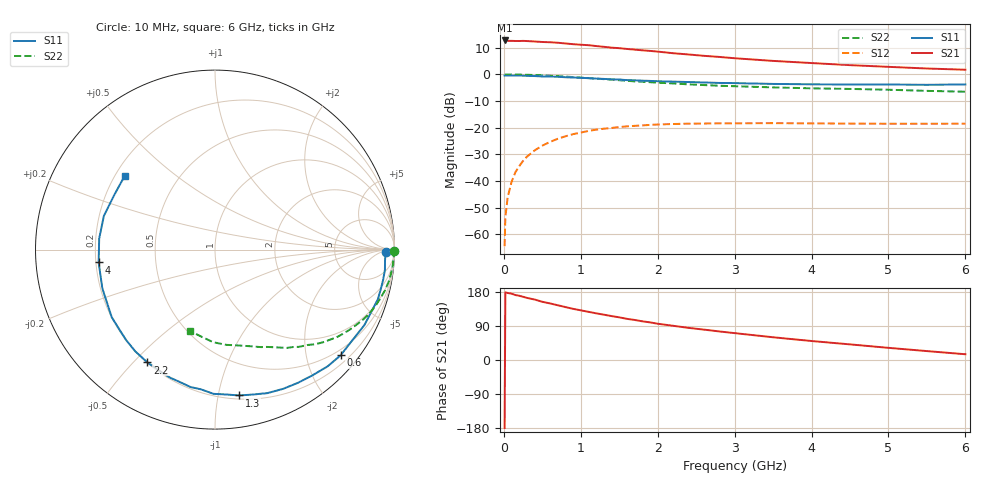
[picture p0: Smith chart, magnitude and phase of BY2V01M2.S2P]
! SIEMENS Small Signal Semiconductors
! BFY420
! Si NPN RF SIEGET Grounded Emitter Transistor in MICRO-X
! VCE = 2 V  IC = 1.2 mA
! Common Emitter S-Parameters:  October  1996
# GHz  S  MA  R  50
!  f  S11  S21  S12  S22
! GHz  MAG  ANG  MAG  ANG  MAG  ANG  MAG  ANG
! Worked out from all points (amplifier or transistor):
!   36 points, 10 MHz to 6 GHz, reference 50 ohm
!   highest |S21| = 12.7 dB at 10 MHz (marker M1)
!   |S21| within 3 dB of that: start of sweep to 1.538 GHz
!   unconditionally stable (mu >= 1): 4.437 GHz to end of sweep
!   at 250 MHz: K = 0.04, MSG = 22.5 dB, |S12| = -32.4 dB
!   at 1.4 GHz: K = 0.22, MSG = 15.1 dB, |S12| = -20.1 dB
!   at 6 GHz: K = 1.32, MAG = 6.8 dB, |S12| = -18.5 dB
!   S11 on the Smith chart (normalised r, x): 10 MHz: 40, -12; 600 MHz: 0.37, -2.69; 1.3 GHz: 0.23, -1.16; 2.2 GHz: 0.20, -0.55; 4 GHz: 0.21, -0.05; 6 GHz: 0.24, +0.34
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0.01  0.9551 -0.8  4.339 -179.4  0.0006 96.0  0.998 -0.3
0.02  0.9498 -1.7  4.339 178.7  0.0021 92.9  0.9928 -0.6
0.05  0.9493 -3.7  4.253 176.8  0.005 85.5  0.9973 -1.7
0.1  0.9534 -6.8  4.266 175.1  0.0096 85.8  0.995 -3.4
0.15  0.9518 -10.2  4.239 171.4  0.0146 81.8  0.9943 -5.1
0.25  0.9486 -17.0  4.26 166.8  0.0239 78.9  0.9884 -8.4
0.4  0.9325 -26.8  4.149 159.6  0.0375 74.0  0.9745 -13.4
0.5  0.9169 -33.5  4.062 153.6  0.0461 70.3  0.9603 -16.5
0.6  0.9146 -40.1  4.015 149.3  0.0542 66.0  0.9459 -19.7
0.8  0.8862 -52.3  3.815 139.7  0.0691 58.4  0.9106 -25.6
1.1  0.8514 -69.9  3.534 127.1  0.0872 49.0  0.8536 -33.3
1.3  0.824 -80.5  3.298 119.6  0.0959 42.9  0.8153 -37.9
1.6  0.7823 -95.8  3.006 108.6  0.1061 35.1  0.7597 -44.1
1.8  0.7636 -104.8  2.833 102.1  0.1106 30.9  0.7285 -47.4
2.2  0.7329 -120.9  2.5 90.3  0.1175 23.2  0.6778 -53.9
2.4  0.7201 -128.1  2.369 84.8  0.1192 20.3  0.6512 -56.9
2.8  0.6927 -141.1  2.13 75.4  0.1211 15.1  0.6134 -62.1
3.5  0.6638 -161.0  1.794 60.0  0.122 8.5  0.5712 -70.4
4  0.6523 -173.7  1.635 50.1  0.1207 5.3  0.5485 -76.7
4.5  0.6482 174.5  1.494 41.2  0.1196 2.6  0.5345 -83.2
5.5  0.6385 151.4  1.292 23.5  0.1187 0.9  0.4916 -98.6
6  0.6494 140.9  1.225 15.2  0.119 1.0  0.4739 -107.4
